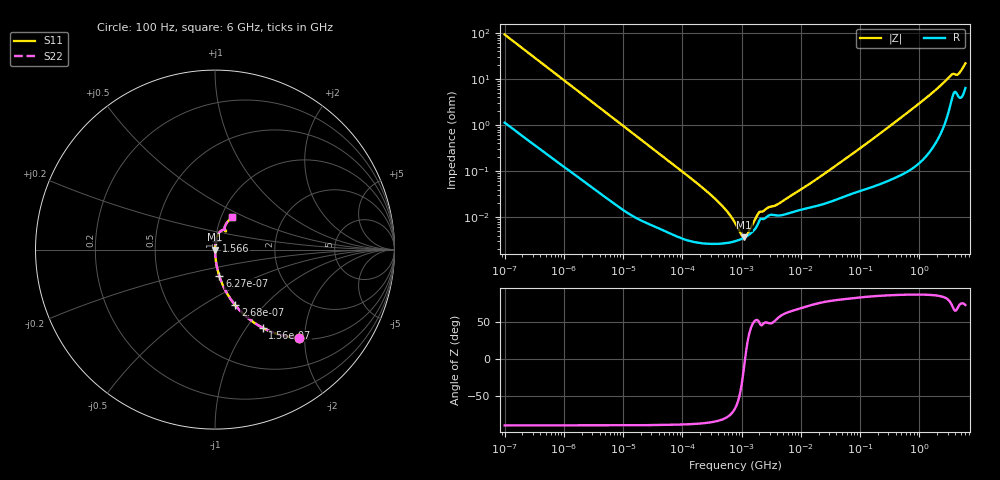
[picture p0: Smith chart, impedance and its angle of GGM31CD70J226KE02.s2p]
!Murata Part Number: GGM31CD70J226KE02
!These Parameters are Measured in Series Mode Connection
!Data Generated on Jun 19, 2026
!  o--ll--o
!Port1  Port2
!  o------o
!Operation Temp=25[degC], DC Bias Voltage=0[V]
!Freq. Start=100[Hz] Stop=6[GHz] 401[Steps]
# Hz S RI R 50
!Freq.(Hz) S11(Real) S11(Imag) S21(Real) S21(Imag) S12(Real) S12(Imag) S22(Real) S22(Imag)
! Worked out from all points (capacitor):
!   401 points, 100 Hz to 6 GHz, reference 50 ohm
!   read as one part in series: C = 17 uF near 109 Hz
!   lowest |Z| = 3.64 mohm at 1.108 MHz (marker M1)
!   series resonance near 1.143 MHz, so ESL is about 1.1 nH
!   S11 on the Smith chart (normalised r, x): 100 Hz: 1.02, -1.86; 156 Hz: 1.01, -1.20; 268 Hz: 1.01, -0.70; 627 Hz: 1.00, -0.30; 1.566 GHz: 1.01, +0.09; 6 GHz: 1.13, +0.42
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100  0.4654 -0.4928  0.5346 0.4928  0.5346 0.4928  0.4654 -0.4928
156  0.266 -0.4358  0.734 0.4358  0.734 0.4358  0.266 -0.4358
268  0.1127 -0.3101  0.8873 0.3101  0.8873 0.3101  0.1127 -0.3101
383  0.0597 -0.2306  0.9403 0.2306  0.9403 0.2306  0.0597 -0.2306
627  0.0241 -0.147  0.9759 0.147  0.9759 0.147  0.0241 -0.147
2008  0.0029 -0.0474  0.9971 0.0474  0.9971 0.0474  0.0029 -0.0474
40335  6.29e-05 -0.00243  0.9999 0.00243  0.9999 0.00243  6.29e-05 -0.00243
231233  2.7e-05 -0.000412  1 0.000412  1 0.000412  2.7e-05 -0.000412
413847  2.65e-05 -0.000208  1 0.000208  1 0.000208  2.65e-05 -0.000208
647581  2.84e-05 -0.000104  1 0.000104  1 0.000104  2.84e-05 -0.000104
774597  3e-05 -6.93e-05  1 6.93e-05  1 6.93e-05  3e-05 -6.93e-05
1108252  3.6e-05 -5.4e-06  1 5.4e-06  1 5.4e-06  3.6e-05 -5.4e-06
1658239  5.4e-05 6.75e-05  0.9999 -6.75e-05  0.9999 -6.75e-05  5.4e-05 6.75e-05
2074311  9.16e-05 9.67e-05  0.9999 -9.67e-05  0.9999 -9.67e-05  9.16e-05 9.67e-05
2837864  0.000108 0.000123  0.9999 -0.000123  0.9999 -0.000123  0.000108 0.000123
4246196  0.000109 0.000165  0.9999 -0.000165  0.9999 -0.000165  0.000109 0.000165
1.555665e7  0.000167 0.000554  0.9998 -0.000554  0.9998 -0.000554  0.000167 0.000554
3.124326e8  0.000718 0.00933  0.9993 -0.00933  0.9993 -0.00933  0.000718 0.00933
1.565993e9  0.00504 0.0469  0.995 -0.0469  0.995 -0.0469  0.00504 0.0469
3.352442e9  0.0389 0.1078  0.9611 -0.1078  0.9611 -0.1078  0.0389 0.1078
4.586474e9  0.053 0.1113  0.947 -0.1113  0.947 -0.1113  0.053 0.1113
6e9  0.0956 0.179  0.9044 -0.179  0.9044 -0.179  0.0956 0.179
